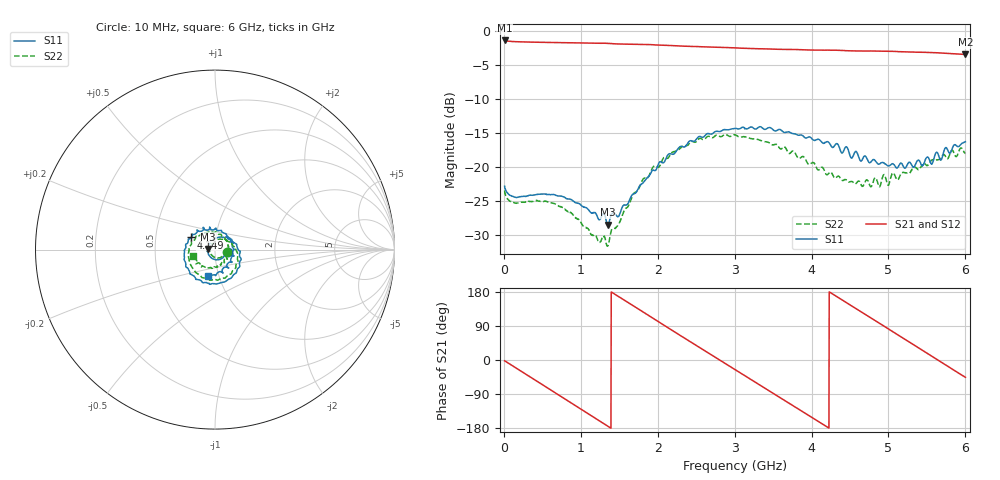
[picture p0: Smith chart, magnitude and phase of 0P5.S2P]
!Agilent Technologies,E5071C,MY46316741,A.11.02
!Date: Thu Jul 30 16:10:15 2020
!Data & Calibration Information:
!Freq	S11:SOLT4(ON)	S21:SOLT4(ON)	S12:SOLT4(ON)	S22:SOLT4(ON)
!PortZ  Port1:50+j0  Port2:50+j0
!Above PortZ is port z conversion or system Z0 setting when saving the data.
!When reading, reference impedance value at option line is always used.
# Hz S dB R 50
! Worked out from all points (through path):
!   1561 points, 10 MHz to 6 GHz, reference 50 ohm
!   highest |S21| = -1.39 dB at 10 MHz (marker M1); lowest = -3.5 dB at 6 GHz (marker M2)
!   group delay of S21, straight-line fit = 354 ps
!   lowest |S11| = -28.5 dB at 1.35 GHz (marker M3), VSWR 1.08, Z = 46.4 + j0.305 ohm
!   |S11| at or under -10 dB: start of sweep to end of sweep
!   |S22| runs from -31.7 to -15.2 dB; largest |S21 - S12| = 0.011
!   S11 on the Smith chart (normalised r, x): 10 MHz: 1.15, -0.03; 4.149 GHz: 0.76, +0.11; 6 GHz: 0.89, -0.27
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1e7  -22.87 -10.9  -1.39 -2.3  -1.39 -2.3  -23.50 -13.5
2.672628e8  -24.36 -19.3  -1.61 -35.1  -1.61 -35.1  -25.22 -19.4
5.514038e8  -24.07 -44.9  -1.68 -71.6  -1.67 -71.7  -25.09 -45.6
7.779487e8  -24.44 -72.2  -1.72 -100.7  -1.72 -100.8  -26.09 -72.6
1.012173e9  -25.77 -109.1  -1.77 -130.8  -1.76 -131.0  -28.44 -111.6
1.350071e9  -28.53 175.0  -1.81 -174.4  -1.81 -174.6  -31.61 150.3
1.65341e9  -24.40 96.1  -1.95 146.8  -1.94 146.5  -24.81 74.5
2.006667e9  -19.68 34.7  -2.08 101.3  -2.07 101.1  -20.10 16.8
2.263929e9  -17.33 -2.9  -2.20 68.5  -2.18 68.1  -17.52 -19.0
2.563429e9  -15.60 -37.4  -2.32 30.5  -2.31 30.2  -15.85 -58.0
2.786135e9  -14.81 -62.9  -2.40 2.3  -2.40 1.8  -15.39 -86.4
3.005e9  -14.36 -86.8  -2.48 -25.5  -2.48 -26.0  -15.29 -115.0
3.266103e9  -14.44 -114.9  -2.60 -58.4  -2.59 -58.9  -15.94 -147.9
3.504167e9  -14.59 -140.3  -2.67 -88.5  -2.66 -89.0  -16.77 179.2
3.742231e9  -15.08 -165.3  -2.72 -118.4  -2.71 -119.0  -17.75 144.6
4.007173e9  -15.91 168.3  -2.80 -151.9  -2.78 -152.6  -19.40 106.9
4.149244e9  -16.54 152.9  -2.82 -169.9  -2.81 -170.5  -20.21 85.9
4.379628e9  -17.75 128.5  -2.86 160.7  -2.85 160.0  -21.81 47.3
4.633051e9  -19.09 98.3  -2.95 128.8  -2.95 128.1  -22.42 8.6
5.001667e9  -19.88 43.1  -2.97 81.7  -2.97 80.9  -22.73 -43.5
5.516192e9  -18.62 -35.7  -3.14 15.9  -3.14 15.1  -19.74 -104.6
6e9  -16.32 -104.6  -3.46 -45.6  -3.44 -46.5  -18.03 -163.6
